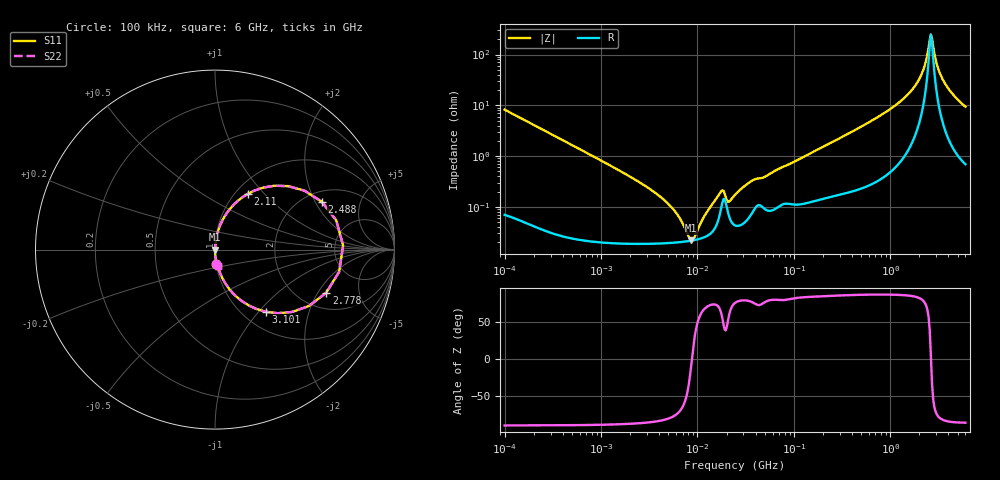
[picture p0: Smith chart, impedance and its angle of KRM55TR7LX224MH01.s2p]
!Murata Part Number: KRM55TR7LX224MH01
!These Parameters are Measured in Series Mode Connection
!Data Generated on Jan 08, 2026
!  o--ll--o
!Port1  Port2
!  o------o
!Operation Temp=25[degC], DC Bias Voltage=0[V]
!Freq. Start=100[kHz] Stop=6[GHz] 401[Steps]
# Hz S RI R 50
!Freq.(Hz) S11(Real) S11(Imag) S21(Real) S21(Imag) S12(Real) S12(Imag) S22(Real) S22(Imag)
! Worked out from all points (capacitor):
!   401 points, 100 kHz to 6 GHz, reference 50 ohm
!   read as one part in series: C = 193 nF near 105.7 kHz
!   lowest |Z| = 21.9 mohm at 8.613 MHz (marker M1)
!   series resonance near 8.758 MHz, so ESL is about 1.7 nH
!   S11 on the Smith chart (normalised r, x): 100 kHz: 1.00, -0.16; 2.11 GHz: 1.14, +0.81; 2.488 GHz: 2.44, +2.27; 2.778 GHz: 2.76, -2.38; 3.101 GHz: 1.26, -1.09; 6 GHz: 1.01, -0.19
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100000  0.0074 -0.0816  0.9926 0.0816  0.9926 0.0816  0.0074 -0.0816
631452  0.00039 -0.013  0.9996 0.013  0.9996 0.013  0.00039 -0.013
3987316  0.000192 -0.00165  0.9998 0.00165  0.9998 0.00165  0.000192 -0.00165
6023672  0.000199 -0.000732  0.9998 0.000732  0.9998 0.000732  0.000199 -0.000732
8612937  0.000216 -3.23e-05  0.9998 3.23e-05  0.9998 3.23e-05  0.000216 -3.23e-05
9353785  0.000223 0.000129  0.9998 -0.000129  0.9998 -0.000129  0.000223 0.000129
1.713112e7  0.000746 0.00173  0.9993 -0.00173  0.9993 -0.00173  0.000746 0.00173
1.860466e7  0.00143 0.00151  0.9986 -0.00151  0.9986 -0.00151  0.00143 0.00151
2.134758e7  0.000638 0.00111  0.9994 -0.00111  0.9994 -0.00111  0.000638 0.00111
2.517799e7  0.000427 0.00178  0.9996 -0.00178  0.9996 -0.00178  0.000427 0.00178
3.700465e7  0.000779 0.00321  0.9992 -0.00321  0.9992 -0.00321  0.000779 0.00321
1.546735e8  0.0014 0.0118  0.9986 -0.0118  0.9986 -0.0118  0.0014 0.0118
9.76689e8  0.0113 0.0809  0.9887 -0.0809  0.9887 -0.0809  0.0113 0.0809
1.693027e9  0.057 0.1903  0.943 -0.1903  0.943 -0.1903  0.057 0.1903
2.10973e9  0.183 0.3107  0.817 -0.3107  0.817 -0.3107  0.183 0.3107
2.355095e9  0.4079 0.3535  0.5921 -0.3535  0.5921 -0.3535  0.4079 0.3535
2.488279e9  0.5947 0.2672  0.4053 -0.2672  0.4053 -0.2672  0.5947 0.2672
2.628996e9  0.7137 0.0221  0.2863 -0.0221  0.2863 -0.0221  0.7137 0.0221
2.77767e9  0.6197 -0.2405  0.3803 0.2405  0.3803 0.2405  0.6197 -0.2405
3.100717e9  0.282 -0.3462  0.718 0.3462  0.718 0.3462  0.282 -0.3462
3.759065e9  0.0831 -0.2237  0.9169 0.2237  0.9169 0.2237  0.0831 -0.2237
6e9  0.0154 -0.0916  0.9846 0.0916  0.9846 0.0916  0.0154 -0.0916
